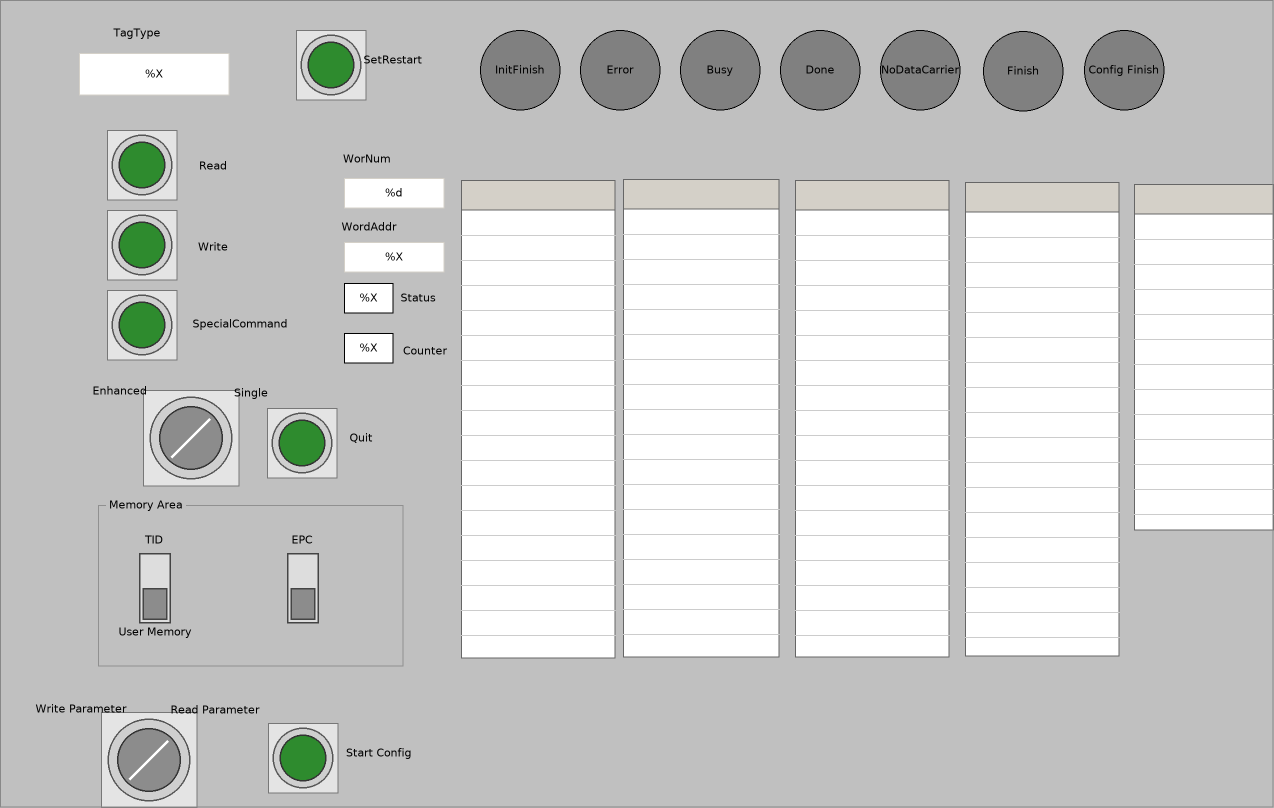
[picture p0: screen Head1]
VISUALIZATION Head1  // 1274x808
    GroupBox (98,497 305x169), "Memory Area"
        DipSwitch (22,56 70x70), variable: MAIN.Head1UserMemoryUID, behaviour: TOGGLE, style: Switch-DipSwitch-Gray
        DipSwitch (170,56 70x70), variable: MAIN.Head1EPC, behaviour: TOGGLE, style: Switch-DipSwitch-Gray
        Label (129,28 150x30), "EPC"
    PushSwitch (107,130 70x70), variable: MAIN.Head1Read, behaviour: TAP, style: Switch-PushSwitch-Green
    PushSwitch (107,210 70x70), variable: MAIN.Head1Write, behaviour: TAP, style: Switch-PushSwitch-Green
    RotarySwitch (138,390 106x96), variable: MAIN.Head1SingleEnhanced, behaviour: TOGGLE, style: Switch-RotarySwitch-Gray
    Textfield (79,53 150x42), "%X", tooltip "TagType", text variable: MAIN.Head1TagType
        OnMouseDown: write MAIN.Head1TagType via Default
    Table (461,180 154x478), data array: MAIN.IC_KP2_2HB21_IQH3_SF_Head1.IDENTControl_FB_SF.INDATA
        p1892666644: MAIN.Data_Channel.InData[2][INDEX]
        p3854506369: MAIN.IC_KP2_2HB21_IQH3_SF_Head1.IDENTControl_FB_SF.INDATA[INDEX]
    Table (623,179 156x478), data array: MAIN.IC_KP2_2HB21_IQH3_SF_Head1.IDENTControl_FB_SF.OUTDATA
        p1892666644: MAIN.Data_Channel.OutData[2][INDEX]
        p3854506369: MAIN.IC_KP2_2HB21_IQH3_SF_Head1.IDENTControl_FB_SF.OUTDATA[INDEX]
        Columns.Column.[0].Template: OnMouseDown: write the text variable via Default
    Textfield (344,242 100x30), "%X", text variable: MAIN.Head1StartAddress
        OnMouseClick: write MAIN.Head1StartAddress via Default
    Textfield (344,178 100x30), "%d", text variable: MAIN.Head1WordNum
        OnMouseClick: write MAIN.Head1WordNum via Default
    PushSwitch (296,30 70x70), variable: MAIN.Head1SetRestart, behaviour: TAP, style: Switch-PushSwitch-Green
    PushSwitch (267,408 70x70), tooltip "Cancel "Enhanced"-Command", variable: MAIN.Head1Quit, behaviour: TAP, style: Switch-PushSwitch-Green
    PushSwitch (107,290 70x70), variable: MAIN.Head1SpecialCommand, behaviour: TAP, style: Switch-PushSwitch-Green
    Table (1134,184 140x346), data array: MAIN.Head1Data.SpecialCommand
        p1892666644: MAIN.Data_Channel.SpecialCommand[2][INDEX]
        p3854506369: MAIN.Head1Data.SpecialCommand[INDEX]
        Columns.Column.[0].Template: OnMouseDown: write the text variable via Default
    Rectangle (344,283 49x30), "%X", text variable: MAIN.Head1Status, input disabled if: TRUE
    Rectangle (344,333 49x30), "%X", text variable: MAIN.Head1ReplyCounter, input disabled if: TRUE
    Ellipse (480,30 80x80), "InitFinish", colour toggle: MAIN.Head1InitFinish
    Ellipse (580,30 80x80), "Error", colour toggle: MAIN.Head1Error
    Ellipse (680,30 80x80), "Busy", colour toggle: MAIN.Head1Busy
    Ellipse (780,30 80x80), "Done", colour toggle: MAIN.Head1Done
    Ellipse (880,30 80x80), "NoDataCarrier", colour toggle: MAIN.Head1NoDataCarrier
    Label (62,18 150x30), "TagType"
    Label (292,144 150x30), "WorNum"
    Label (294,212 150x30), "WordAddr"
    Label (343,283 150x30), "Status"
    Label (350,336 150x30), "Counter"
    Label (138,151 150x30), "Read"
    Label (138,232 150x30), "Write"
    Label (165,309 150x30), "SpecialCommand"
    Label (45,376 150x30), "Enhanced"
    Label (176,378 150x30), "Single"
    Label (286,423 150x30), "Quit"
    Label (79,525 150x30), "TID"
    Label (80,617 150x30), "User Memory"
    Ellipse (983,31 80x80), "Finish", colour toggle: MAIN.Head1Finish
    Table (795,180 154x477), data array: MAIN.Head1Data.ReadData
        p1892666644: MAIN.Data_Channel.SpecialCommand[2][INDEX]
        p3854506369: MAIN.Head1Data.ReadData[INDEX]
        Columns.Column.[0].Template: OnMouseDown: write the text variable via Default
    Table (965,182 154x474), data array: MAIN.Head1Data.WriteData
        p1892666644: MAIN.Data_Channel.SpecialCommand[2][INDEX]
        p3854506369: MAIN.Head1Data.WriteData[INDEX]
        Columns.Column.[0].Template: OnMouseDown: write the text variable via Default
    Label (318,45 150x30), "SetRestart"
    RotarySwitch (96,712 106x96), variable: MAIN.Head1WriteParameter, behaviour: TOGGLE, style: Switch-RotarySwitch-Gray
    Label (140,695 150x30), "Read Parameter"
    Label (6,694 150x30), "Write Parameter"
    PushSwitch (268,723 70x70), variable: MAIN.Head1StartConfig, behaviour: TAP, style: Switch-PushSwitch-Green
    Label (304,739 150x28), "Start Config"
    Ellipse (1084,30 80x80), "Config Finish", colour toggle: MAIN.Head1EndConfig
END_VISUALIZATION
